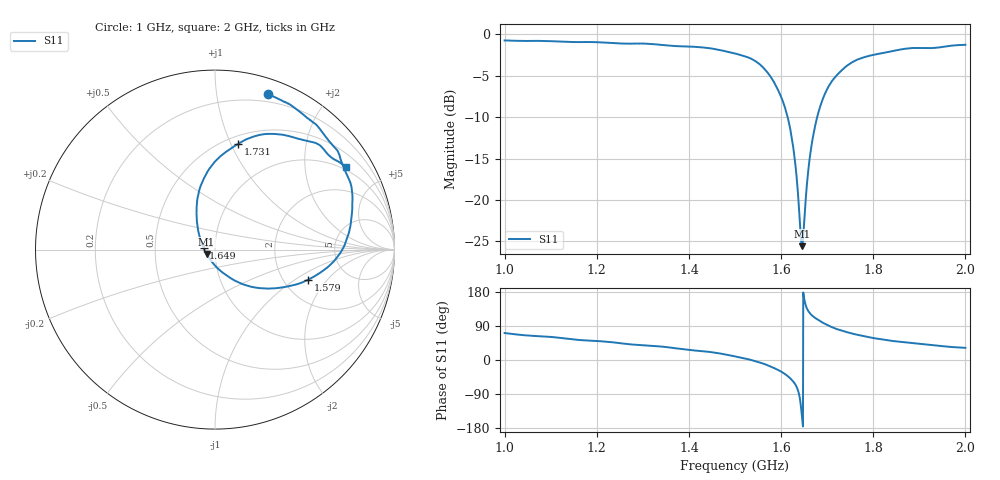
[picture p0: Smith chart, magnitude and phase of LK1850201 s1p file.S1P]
!Agilent Technologies,E5071C,
!Date: Fri Sep 29 19:37:18 2023
!Data & Calibration Information:
!Freq	S11:SOLT1(ON)
!PortZ  Port1:50+j0
!Above PortZ is port z conversion or system Z0 setting when saving the data.
!When reading, reference impedance value at option line is always used.
# Hz S RI R 50
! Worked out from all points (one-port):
!   1601 points, 1 GHz to 2 GHz, reference 50 ohm
!   lowest |S11| = -25.6 dB at 1.646 GHz (marker M1), VSWR 1.11, Z = 45.5 - j2.16 ohm
!   |S11| at or under -10 dB: 1.614 GHz to 1.678 GHz (64.1 MHz wide, 3.89 % of centre)
!   S11 on the Smith chart (normalised r, x): 1 GHz: 0.13, +1.39; 1.579 GHz: 2.71, -1.29; 1.649 GHz: 0.88, +0.02; 1.731 GHz: 0.58, +1.07; 2 GHz: 0.91, +3.24
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1e9  0.2953 0.8665
1.045625e9  0.3831 0.8244
1.125e9  0.4804 0.7611
1.16375e9  0.544 0.7106
1.25e9  0.627 0.6156
1.330625e9  0.696 0.5156
1.375e9  0.7302 0.4271
1.4475e9  0.7662 0.293
1.5e9  0.7532 0.1262
1.54375e9  0.6882 -0.0329
1.57875e9  0.5194 -0.1676
1.6075e9  0.2963 -0.2173
1.616875e9  0.2075 -0.2083
1.625e9  0.1268 -0.1805
1.633125e9  0.0505 -0.1342
1.641875e9  -0.0229 -0.0612
1.645625e9  -0.0471 -0.0237
1.64875e9  -0.0634 0.00862
1.656875e9  -0.0912 0.0946
1.661875e9  -0.0994 0.1458
1.66875e9  -0.1029 0.2128
1.6775e9  -0.0959 0.2942
1.7e9  -0.0201 0.4658
1.73125e9  0.1301 0.5895
1.75e9  0.215 0.6296
1.806875e9  0.4172 0.6309
1.875e9  0.5683 0.5906
2e9  0.7305 0.4583
